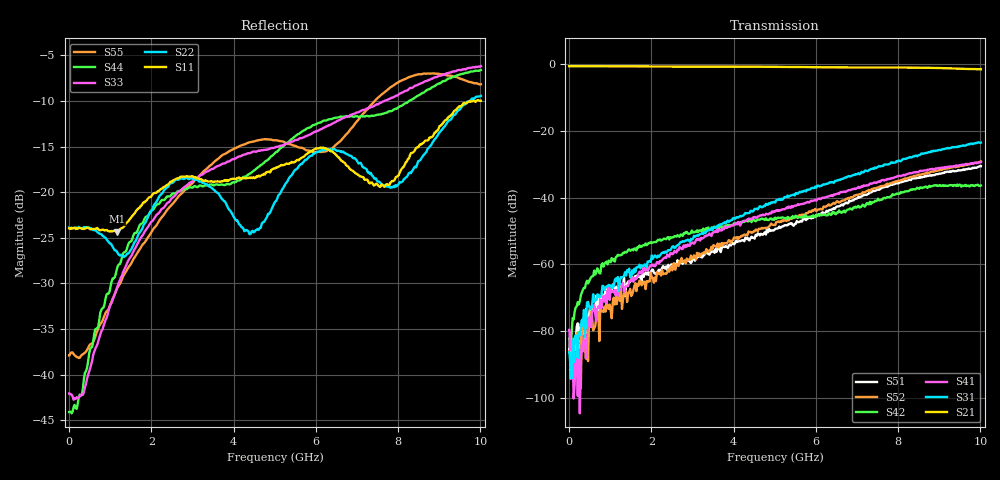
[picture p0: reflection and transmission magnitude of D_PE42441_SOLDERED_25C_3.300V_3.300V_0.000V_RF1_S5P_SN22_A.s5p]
! Device ID: PE42441
! Serial: 22
! Insertion: A
! Temp: 25C
! VDD: 3.300
! Control_Hi: 100.000
! Control_Lo: 0.000
! Logic State: RF1
! Port 1: RFC
! Port 2: RF1
! Port 3: RF2
! Port 4: RF3
! Port 5: RF4
! V1 = 0.00
! V2 = 0.00
! V3 = 0.00
! V4 = 0.00
! IDD: 1.118274e-04
! 1 Hz data is simulated
#  Hz  S  RI  R  50
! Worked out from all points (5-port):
!   402 points, 1 Hz to 10.01 GHz, reference 50 ohm
!   strongest paths, dB at 1 Hz, 2.485 GHz, 5.01 GHz, 7.51 GHz, 10.01 GHz:
!     S21: -0.7, -0.8, -0.8, -1.0, -1.6
!     S31: -86.3, -55.3, -41.5, -30.8, -23.5
!     S41: -79.6, -56.7, -44.2, -35.3, -29.4
!     S42: -82.2, -52.0, -46.0, -40.3, -36.4
!     S52: -85.9, -60.6, -48.3, -37.0, -29.1
!     S51: -85.6, -60.0, -49.4, -37.6, -30.6
!   lowest |S11| = -24.3 dB at 1.16 GHz (marker M1), VSWR 1.13, Z = 54.4 - j4.59 ohm
!   |S11| at or under -10 dB: start of sweep to 9.819 GHz; 9.844 GHz to 9.9 GHz (56.39 MHz wide, 0.571 % of centre)
